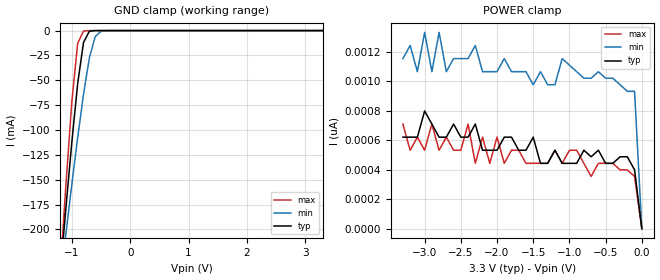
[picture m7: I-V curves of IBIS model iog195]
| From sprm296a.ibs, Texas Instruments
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[Model]   iog195
Model_type   Terminator
Polarity   Non-Inverting
| signals   Y
|   typ   min   max
C_comp   3.670p   3.531p   3.708p
|   typ   min   max
[Temperature Range]   25   -40   125
|   typ   min   max
[Voltage Range]   3.30V   3.00V   3.60V
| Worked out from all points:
|   GND clamp passes 1 mA (typ) near -0.70 V on its own axis
[GND_clamp]
|   Voltage   I(typ)   I(min)   I(max)
-3.3V     -1.775A    -1.357A    -2.276A
-1.2V     -245.6mA   -253.2mA   -243.1mA
-1.1V     -177.5mA   -203.4mA   -153.8mA
-1V       -112.2mA   -154.6mA   -71.62mA
-900mV    -53.36mA   -107.7mA   -12.89mA
-800mV    -12.02mA   -64.09mA   -440.6uA
-700mV    -680.2uA   -27.6mA    -16.59uA
-600mV    -25.98uA   -6.116mA   -517.1nA
-500mV    -911.2nA   -578.8uA   -11.12nA
3.3V      355.3pA    977pA      399.7pA
[POWER_clamp]
|   Voltage   I(typ)   I(min)   I(max)
-3.3V     621.7pA    1.155nA    710.5pA
-3.1V     621.7pA    1.066nA    621.7pA
-3V       799.4pA    1.332nA    532.9pA
-2.9V     710.5pA    1.066nA    710.5pA
-2.8V     621.7pA    1.332nA    532.9pA
-2.7V     621.7pA    1.066nA    621.7pA
-2.4V     621.7pA    1.155nA    710.5pA
-2.3V     710.5pA    1.243nA    444.1pA
-2V       532.9pA    1.066nA    621.7pA
-1.9V     621.7pA    1.155nA    444.1pA
-100mV    399.7pA    932.6pA    355.3pA
0V        1pA        1pA        1pA
